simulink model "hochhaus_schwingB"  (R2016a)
settings: Solver=ode45  StartTime=0.0  StopTime=400  RelTol=1e-3
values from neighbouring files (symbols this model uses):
  m = 1.0    (= 1)    [init_pendelStange.m]
undefined symbols (not defined in the file or in its folder): v0, x0
libraries: simulink_extras x2

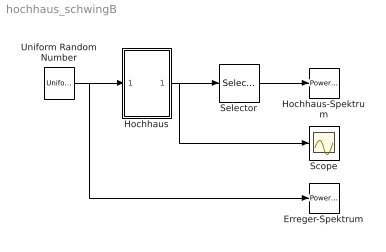
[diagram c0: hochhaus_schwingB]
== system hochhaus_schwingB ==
  Erreger-Spektrum : simulink_extras/Additional Sinks/Power Spectral Density  npts=2048  fftpts=2048  HowOften=64  sampleT=0.05
  Hochhaus : Subsystem
  Hochhaus-Spektrum : simulink_extras/Additional Sinks/Power Spectral Density  npts=2048  fftpts=2048  HowOften=64  sampleT=0.05
  Scope : Scope
  Selector : Selector  InputPortWidth=3  IndexOptions=Index vector (dialog)  Indices=[1]  OutputSizes=1
  Uniform Random Number : UniformRandomNumber  SampleTime=0.05
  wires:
  Hochhaus/1(x) -> Selector/1, Scope/1
  Uniform Random Number/1 -> Hochhaus/1(F), Erreger-Spektrum/1
  Selector/1 -> Hochhaus-Spektrum/1

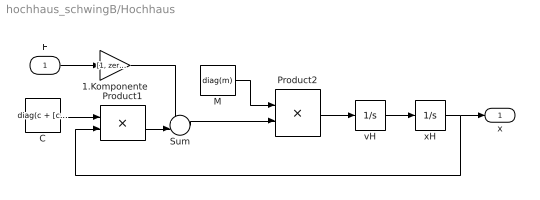
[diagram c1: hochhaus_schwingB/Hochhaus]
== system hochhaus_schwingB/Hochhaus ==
  F : Inport
  1.Komponente : Gain  Gain=[1, zeros(1,length(m)-1)]
  C : Constant  Value=diag(c + [c(2:end),0]) - diag(c(2:end),1) - diag(c(2:end),-1)  VectorParams1D=off
  M : Constant  Value=diag(m)  VectorParams1D=off
  Product1 : Product  Multiplication=Matrix(*)
  Product2 : Product  Inputs=/*  Multiplication=Matrix(*)
  Sum : Sum  Inputs=+-|
  vH : Integrator  InitialCondition=v0
  xH : Integrator  InitialCondition=x0
  x : Outport
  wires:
  1.Komponente/1 -> Sum/1
  F/1 -> 1.Komponente/1
  M/1 -> Product2/1
  Product2/1 -> vH/1
  Sum/1 -> Product2/2
  C/1 -> Product1/1
  Product1/1 -> Sum/2
  xH/1 -> x/1, Product1/2
  vH/1 -> xH/1
